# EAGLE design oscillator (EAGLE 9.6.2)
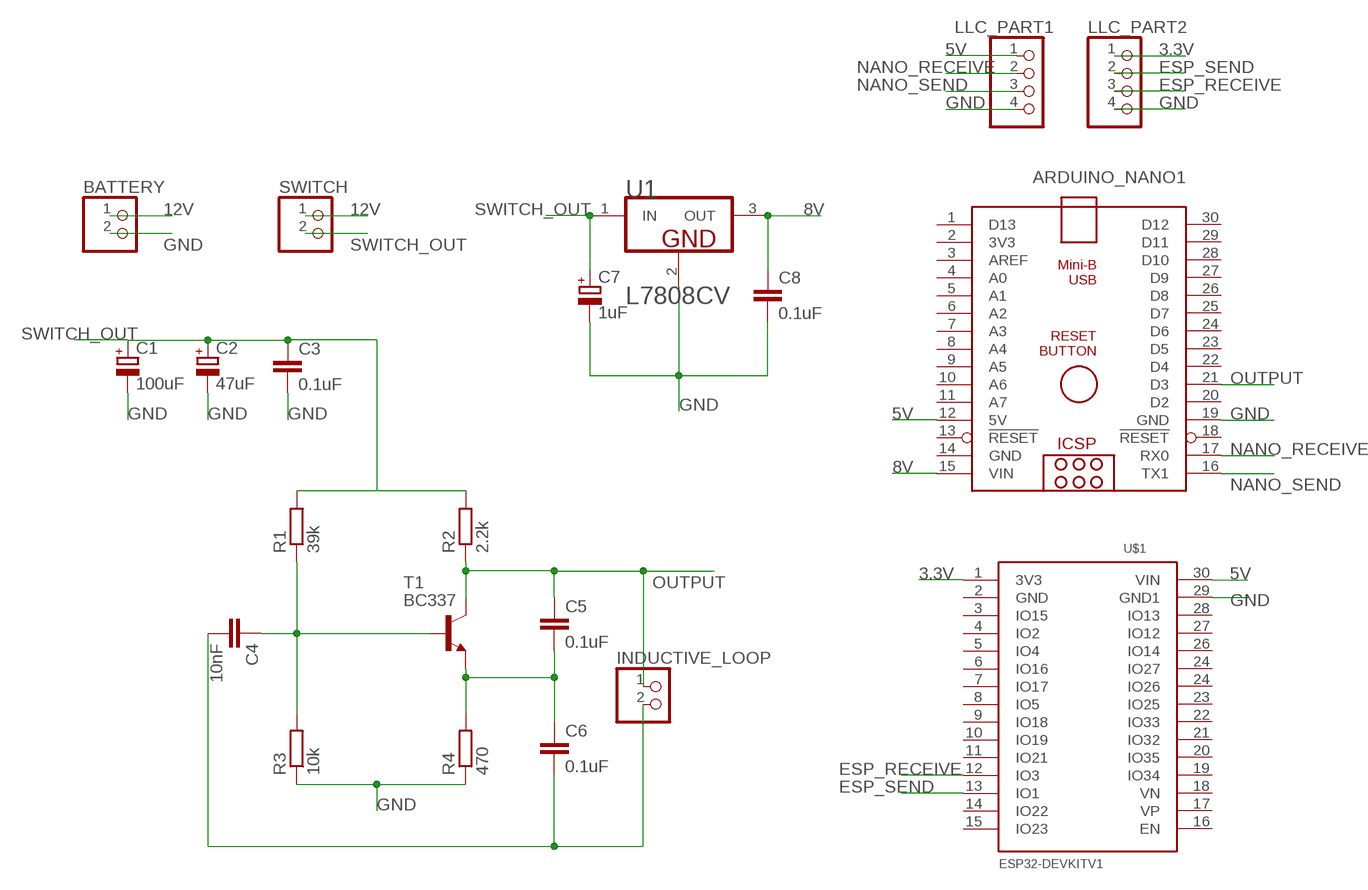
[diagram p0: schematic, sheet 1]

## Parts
ARDUINO_NANO1  ARDUINO_NANO  [ARDUINO_NANO]
BATTERY  PINHD-1X2  [1X02]
C1  100uF  CPOL-EUE2,5-6E  [E2,5-6E]
C2  47uF  CPOL-EUE2,5-6E  [E2,5-6E]
C3  0.1uF  C-EU025-025X050  [C025-025X050]
C4  10nF  C-EU025-025X050  [C025-025X050]
C5  0.1uF  C-EU225-087X268  [C225-087X268]
C6  0.1uF  C-EU225-087X268  [C225-087X268]
C7  1uF  CPOL-EUE2,5-6E  [E2,5-6E]
C8  0.1uF  C-EU025-025X050  [C025-025X050]
INDUCTIVE_LOOP  PINHD-1X2  [1X02]
LLC_PART1  PINHD-1X4  [1X04]
LLC_PART2  PINHD-1X4  [1X04]
R1  39k  R-EU_0207/10  [0207/10]
R2  2.2k  R-EU_0207/10  [0207/10]
R3  10k  R-EU_0207/10  [0207/10]
R4  470  R-EU_0207/10  [0207/10]
SWITCH  PINHD-1X2  [1X02]
T1  BC337  [TO92]
U1  STMICROELECTRONICS_L7808CVSTMICROELECTRONICS_L7808CV_0_0  [STMICROELECTRONICS_L7808CV_0]
U$1  ESP32DEVKITV1  [ESP32-DEVKITV1]

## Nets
3.3V: LLC_PART2.1 U$1.1(3V3)
5V: ARDUINO_NANO1.12(5V) LLC_PART1.1 U$1.30(VIN)
8V: ARDUINO_NANO1.15(VIN) C8.1 U1.3(OUT)
12V: BATTERY.1 SWITCH.1
ESP_RECEIVE: LLC_PART2.3 U$1.12(IO3)
ESP_SEND: LLC_PART2.2 U$1.13(IO1)
GND: ARDUINO_NANO1.19(GND) BATTERY.2 C1.- C2.- C3.2 C7.- C8.2 LLC_PART1.4 LLC_PART2.4 R3.1 R4.1 U1.2(GND) U$1.29(GND1)
LOOP_END2: C4.2 C6.2 INDUCTIVE_LOOP.2
N$3: C5.2 C6.1 R4.2 T1.1(E)
N$4: C4.1 R1.1 R3.2 T1.2(B)
NANO_RECEIVE: ARDUINO_NANO1.17(RX0) LLC_PART1.2
NANO_SEND: ARDUINO_NANO1.16(TX1) LLC_PART1.3
OUTPUT: ARDUINO_NANO1.21(D3) C5.1 INDUCTIVE_LOOP.1 R2.1 T1.3(C)
SWITCH_OUT: C1.+ C2.+ C3.1 C7.+ R1.2 R2.2 SWITCH.2 U1.1(IN)
Unconnected: ARDUINO_NANO1.1(D13) ARDUINO_NANO1.2(3V3) ARDUINO_NANO1.3(AREF) ARDUINO_NANO1.4(A0) ARDUINO_NANO1.5(A1) ARDUINO_NANO1.6(A2) ARDUINO_NANO1.7(A3) ARDUINO_NANO1.8(A4) ARDUINO_NANO1.9(A5) ARDUINO_NANO1.10(A6) ARDUINO_NANO1.11(A7) ARDUINO_NANO1.13(!RESET) ARDUINO_NANO1.18(!RESET) ARDUINO_NANO1.20(D2) ARDUINO_NANO1.22(D4) ARDUINO_NANO1.23(D5) ARDUINO_NANO1.24(D6) ARDUINO_NANO1.25(D7) ARDUINO_NANO1.26(D8) ARDUINO_NANO1.27(D9) ARDUINO_NANO1.28(D10) ARDUINO_NANO1.29(D11) ARDUINO_NANO1.30(D12) U$1.2(GND) U$1.3(IO15) U$1.4(IO2) U$1.5(IO4) U$1.6(IO16) U$1.7(IO17) U$1.8(IO5) U$1.9(IO18) U$1.10(IO19) U$1.11(IO21) U$1.14(IO22) U$1.15(IO23) U$1.16(EN) U$1.17(VP) U$1.18(VN) U$1.19(IO34) U$1.20(IO35) U$1.21(IO32) U$1.22(IO33) U$1.23(IO25) U$1.24(IO26) U$1.24(IO27) U$1.26(IO14) U$1.27(IO12) U$1.28(IO13)

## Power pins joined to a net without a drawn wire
GND: ARDUINO_NANO1.14(GND)

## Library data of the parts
ARDUINO_NANO1 = ArduinoNanoV30:ARDUINO_NANO: Arduino Nano V3.0 Overview: The Arduino Nano is a small, complete, and breadboard-friendly board based on the ATmega328 (Arduino Nano 3.x) or ATmega168 (Arduino Nano 2.x). It has more or less the same functionality of the Arduino Duemilanove, but in a different package. It lacks only a DC power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
BATTERY INDUCTIVE_LOOP SWITCH = pinhead:PINHD-1X2: PIN HEADER
C1 C2 C7 = rcl:CPOL-EU: POLARIZED CAPACITOR, European symbol; SPICEPREFIX: C
C3-C6 C8 = rcl:C-EU: CAPACITOR, European symbol; SPICEPREFIX: C
LLC_PART1 LLC_PART2 = pinhead:PINHD-1X4: PIN HEADER
R1-R4 = rcl:R-EU_: RESISTOR, European symbol; SPICEPREFIX: R
T1 = transistor:BC337: NPN TRANSISTOR
U1 = STMicroelectronics - L7808CV:STMICROELECTRONICS_L7808CV: PM-REG-L4940-SIL3; CIIVA_IDS: 1170723; COMPONENT_LINK_1_DESCRIPTION: Manufacturer URL; COMPONENT_LINK_1_URL: http://www.st.com; COMPONENT_LINK_3_DESCRIPTION: Package Specification; COMPONENT_LINK_3_URL: http://www.st.com/internet/com/TECHNICAL_RESOURCES/TECHNICAL_LITERATURE/PACKAGE_INFORMATION/CD00004649.pdf; DATASHEET: http://www.st.com/internet/com/TECHNICAL_RESOURCES/TECHNICAL_LITERATURE/DATASHEET/CD00000444.pdf; DATASHEET_VERSION: 16/11/2011; FOOTPRINT_VARIANT_NAME_0: Manufacturer Recommended; IMPORTED: yes; IMPORTED_FROM: vault; IMPORT_TS: 1521848887; MF: STMicroelectronics; MPN: L7808CV; PACKAGE: TO220; PACKAGE_DESCRIPTION: TO, Thru-Hole, Vertical, Heatsink Mounted; 3 In-Line Leads; Pitch 2.54 mm; PACKAGE_VERSION: ver3.0; PREFIX: U; RELEASE_DATE: 1329864171; VAULT_GUID: 7E0061DC-0552-4B91-9AF1-2862D70182D9; VAULT_REVISION: A0271135-C66A-4FB1-B3B8-70AD1277C65C
U$1 = ESP32-DEVKITV1:ESP32DEVKITV1

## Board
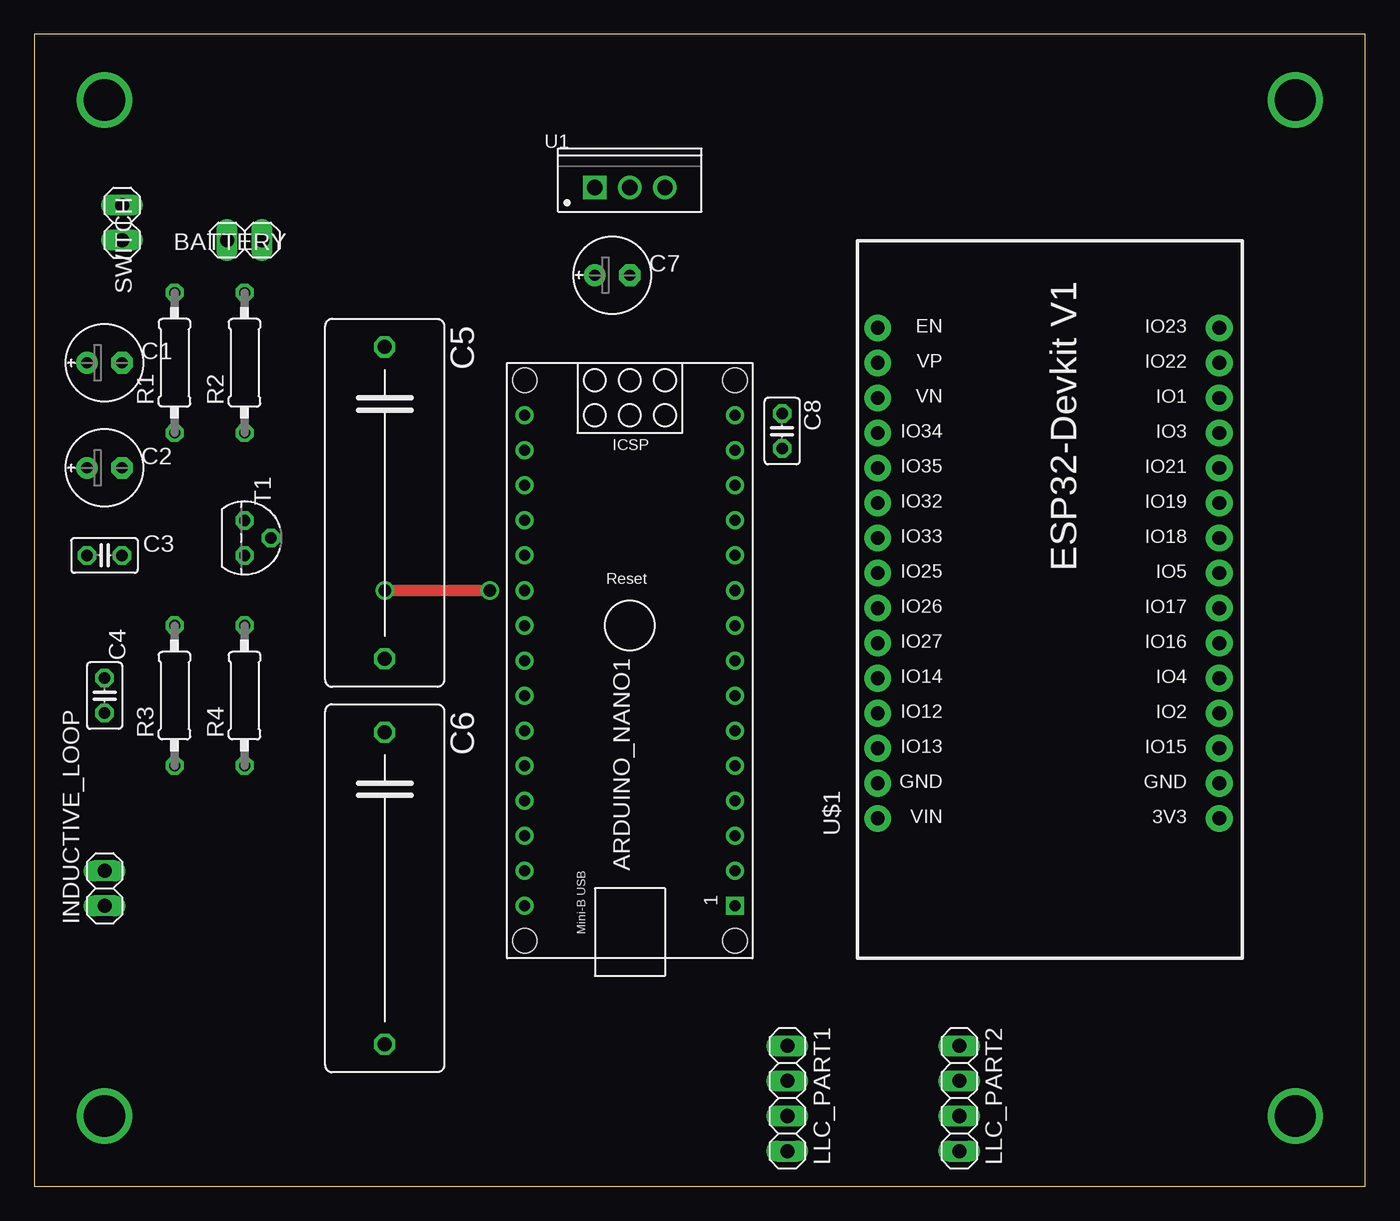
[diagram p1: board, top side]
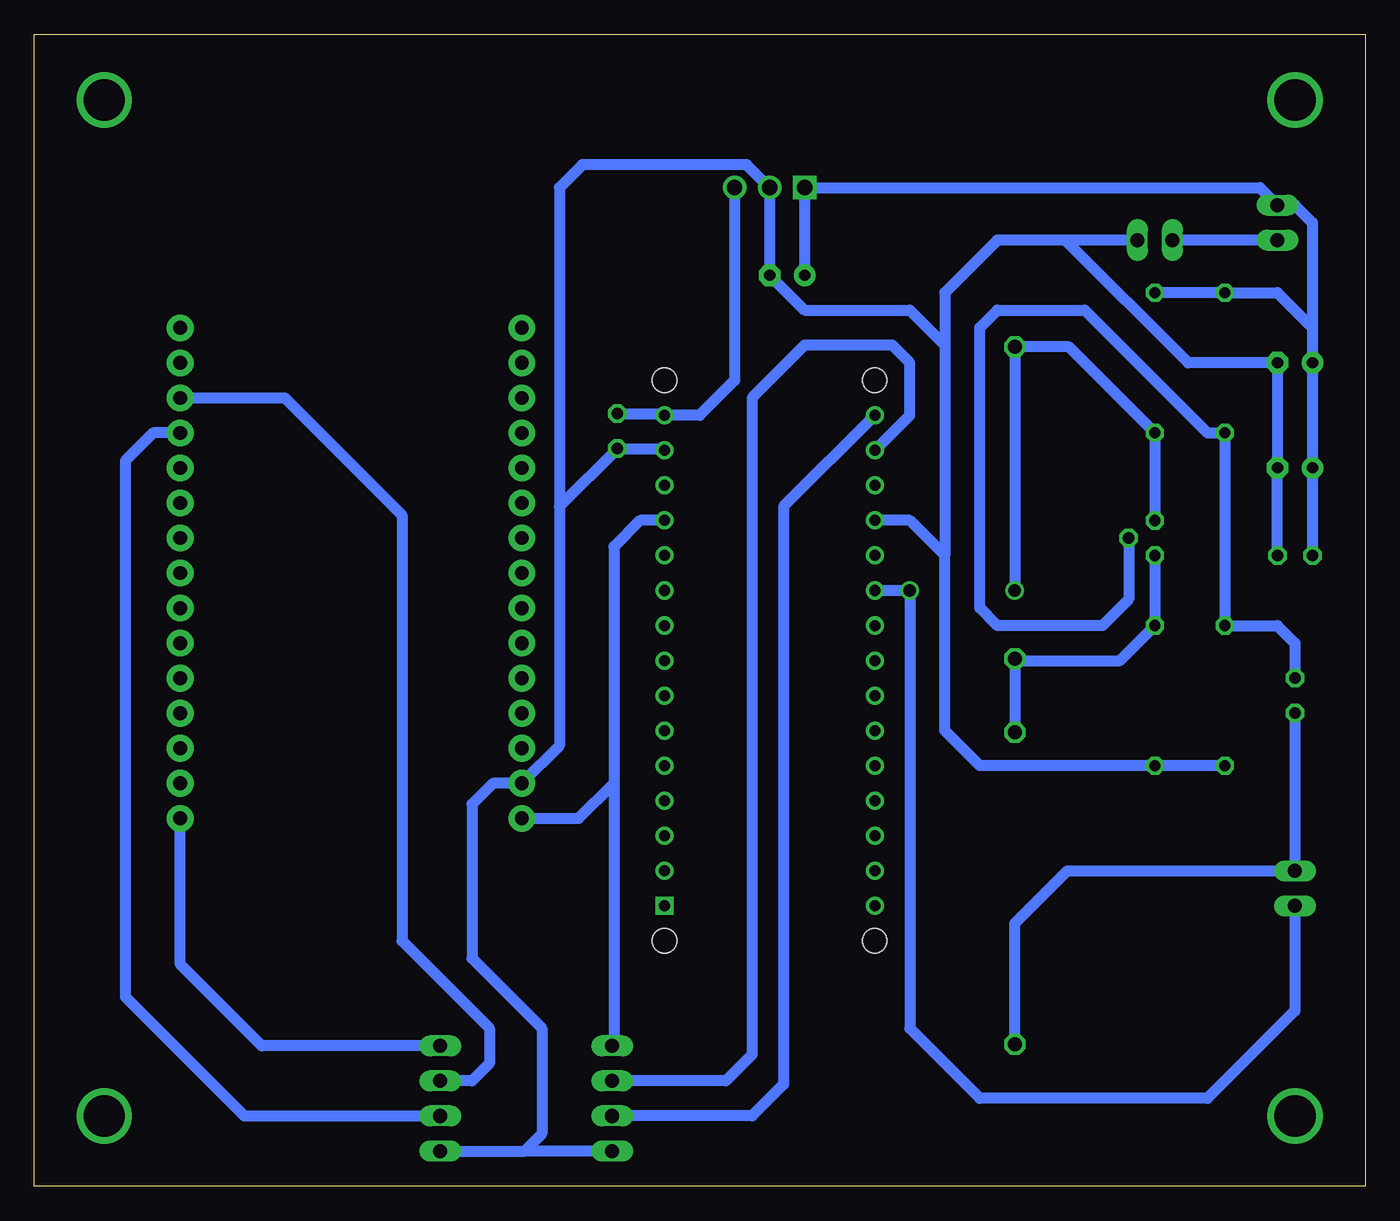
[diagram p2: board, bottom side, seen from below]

Size 96.5 x 83.49 mm. Coordinates in mm from the lower left corner, seen from the top.
Outline: 0,0 96.5,0 96.5,83.49 0,83.49 0,0
Copper layers (1*16): Top 0.035mm / dielectric 1.5mm / Bottom 0.035mm
Design rules "default *": minimum track width 6mil, minimum drill 0.35mm, track to track 16mil, track to pad 16mil, pad to pad 16mil, via to via 16mil, smd to smd 16mil, copper to edge 40mil, drill to drill 6mil, minimum pad ring 10mil, minimum via ring 8mil, stop-mask expansion 4mil, vias tented up to drill 0mil, thermal gap 10mil

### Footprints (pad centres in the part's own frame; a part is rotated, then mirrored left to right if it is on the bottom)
ARDUINO_NANO = drill 0.8 square: 1 -20.32,-7.62 | drill 0.8: 2 -17.78,-7.62; 3 -15.24,-7.62; 4 -12.7,-7.62; 5 -10.16,-7.62; 6 -7.62,-7.62; 7 -5.08,-7.62; 8 -2.54,-7.62; 9 0,-7.62; 10 2.54,-7.62; 11 5.08,-7.62; 12 7.62,-7.62; 13 10.16,-7.62; 14 12.7,-7.62; 15 15.24,-7.62; 16 15.24,7.62; 17 12.7,7.62; 18 10.16,7.62; 19 7.62,7.62; 20 5.08,7.62; 21 2.54,7.62; 22 0,7.62; 23 -2.54,7.62; 24 -5.08,7.62; 25 -7.62,7.62; 26 -10.16,7.62; 27 -12.7,7.62; 28 -15.24,7.62; 29 -17.78,7.62; 30 -20.32,7.62 | hole 1.778: -22.86,-7.62; -22.86,7.62; 17.78,7.62; 17.78,-7.62
1X02 = drill 1.016 long: 1 -1.27,0; 2 1.27,0
E2,5-6E = drill 0.813 pad 1.575: + -1.27,0 | drill 0.813 pad 1.575 octagon: - 1.27,0
C025-025X050 = drill 0.813 octagon: 1 -1.27,0; 2 1.27,0
C225-087X268 = drill 1.016 octagon: 1 -11.303,0; 2 11.303,0
1X04 = drill 1.016 long: 1 -3.81,0; 2 -1.27,0; 3 1.27,0; 4 3.81,0
0207/10 = drill 0.813 octagon: 1 -5.08,0; 2 5.08,0
TO92 = drill 0.813 octagon: 1 1.27,0; 2 0,1.905; 3 -1.27,0
STMICROELECTRONICS_L7808CV_0 = drill 1.1 pad 1.7 square: 1 -2.54,0 | drill 1.1 pad 1.7: 2 0,0; 3 2.54,0
ESP32-DEVKITV1 = drill 1 pad 1.93: 1 -22.87,-13.54; 2 -20.33,-13.54; 3 -17.79,-13.54; 4 -15.25,-13.54; 5 -12.71,-13.54; 6 -10.17,-13.54; 7 -7.63,-13.54; 8 -5.09,-13.54; 9 -2.55,-13.54; 10 -0.01,-13.54; 11 2.53,-13.54; 12 5.07,-13.54; 13 7.61,-13.54; 14 10.15,-13.54; 15 12.69,-13.54; 16 12.69,11.23; 17 10.15,11.23; 18 7.61,11.23; 19 5.07,11.23; 20 2.53,11.23; 21 -0.01,11.23; 22 -2.55,11.23; 23 -5.09,11.23; 24 -7.63,11.23; 25 -10.17,11.23; 26 -12.71,11.23; 27 -15.25,11.23; 28 -17.79,11.23; 29 -20.33,11.23; 30 -22.87,11.23

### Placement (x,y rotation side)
ARDUINO_NANO1  43.18,40.64 90 top
BATTERY  15.24,68.58 0 top
C1  5.08,59.69 0 top
C2  5.08,52.07 0 top
C3  5.08,45.72 0 top
C4  5.08,35.56 270 top
C5  25.4,49.53 270 top
C6  25.4,21.59 270 top
C7  41.91,66.04 0 top
C8  54.23,54.74 270 top
INDUCTIVE_LOOP  5.08,21.59 90 top
LLC_PART1  54.61,6.35 270 top
LLC_PART2  67.07,6.35 270 top
R1  10.16,59.69 90 top
R2  15.24,59.69 90 top
R3  10.16,35.56 90 top
R4  15.24,35.56 90 top
SWITCH  6.35,69.85 90 top
T1  15.24,46.99 270 top
U1  43.18,72.39 0 top
U$1  72.39,49.53 90 top

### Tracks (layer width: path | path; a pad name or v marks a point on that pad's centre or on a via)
3.3V
  Bottom 0.813: U$1.1 85.93,16.08 80.01,10.16 LLC_PART2.1
5V
  Bottom 0.813: ARDUINO_NANO1.12 52.58,48.26 54.48,46.36 54.48,29.21 | LLC_PART1.1 54.48,10.29 54.48,29.21 | U$1.30 57.03,26.66 54.48,29.21
8V
  Bottom 0.813: C8.1 50.93,56.01 ARDUINO_NANO1.15 48.26,55.88 45.72,58.42 U1.3
12V
  Bottom 0.813: SWITCH.1 BATTERY.1
ESP_RECEIVE
  Bottom 0.813: U$1.12 87.89,54.6 89.92,52.58 89.92,13.72 81.28,5.08 LLC_PART2.3
ESP_SEND
  Bottom 0.813: U$1.13 78.35,57.14 69.85,48.64 69.85,17.78 63.5,11.43 63.5,8.89 64.77,7.62 LLC_PART2.2
GND
  Bottom 0.813: R3.1 R4.1 27.94,30.48 30.48,33.02 30.48,45.72 | 30.48,45.72 33.02,48.26 ARDUINO_NANO1.19 | ARDUINO_NANO1.14 50.93,53.47 C8.2 58.42,49.28 | 58.42,49.28 58.42,31.94 U$1.29 63.26,29.2 64.77,27.69 64.77,16.51 59.69,11.43 59.69,3.81 60.96,2.54 | 58.42,49.28 58.42,72.39 56.76,74.05 44.84,74.05 U1.2 C7.- 40.64,63.5 33.02,63.5 30.48,60.96 | C3.2 C2.- C1.- 12.83,59.69 21.72,68.58 | 30.48,60.96 30.48,64.77 26.67,68.58 21.72,68.58 | 30.48,60.96 30.48,45.72 | LLC_PART2.4 60.96,2.54 | LLC_PART1.4 60.96,2.54 | BATTERY.2 21.72,68.58
LOOP_END2
  Bottom 0.813: C4.2 INDUCTIVE_LOOP.2 21.59,22.86 25.4,19.05 C6.2
N$1  (via drill 3)
  other vias: 5.08,78.74
N$2  (via drill 3)
  other vias: 91.44,78.74
N$3
  Bottom 0.813: C6.1 C5.2 25.27,38.1 17.78,38.1 R4.2 T1.1
N$4
  Bottom 0.813: C4.1 5.08,39.37 6.35,40.64 R3.2 R1.1 11.43,54.61 20.32,63.5 26.67,63.5 27.94,62.23 27.94,41.91 26.67,40.64 19.05,40.64 17.14,42.55 T1.2
N$5  (via drill 3)
  other vias: 91.44,5.08
N$6  (via drill 3)
  other vias: 5.08,5.08
NANO_RECEIVE
  Bottom 0.813: ARDUINO_NANO1.17 33.02,55.88 33.02,59.69 34.29,60.96 40.64,60.96 44.45,57.15 44.45,9.52 46.35,7.62 LLC_PART1.2
NANO_SEND
  Bottom 0.813: ARDUINO_NANO1.16 42.16,49.28 42.16,7.37 44.45,5.08 LLC_PART1.3
OUTPUT  (via drill 0.9)
  Top 0.813: v25.4,43.18 v33.02,43.18
  Bottom 0.813: T1.3 R2.1 21.46,60.83 C5.1 v25.4,43.18 | INDUCTIVE_LOOP.1 5.08,12.7 11.43,6.35 27.94,6.35 33.02,11.43 v33.02,43.18 ARDUINO_NANO1.21
SWITCH_OUT
  Bottom 0.813: R2.2 R1.2 6.35,64.77 3.81,62.23 | C3.1 C2.+ C1.+ 3.81,62.23 | 3.81,62.23 3.81,69.85 5.08,71.12 SWITCH.2 7.62,72.39 U1.1 C7.+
